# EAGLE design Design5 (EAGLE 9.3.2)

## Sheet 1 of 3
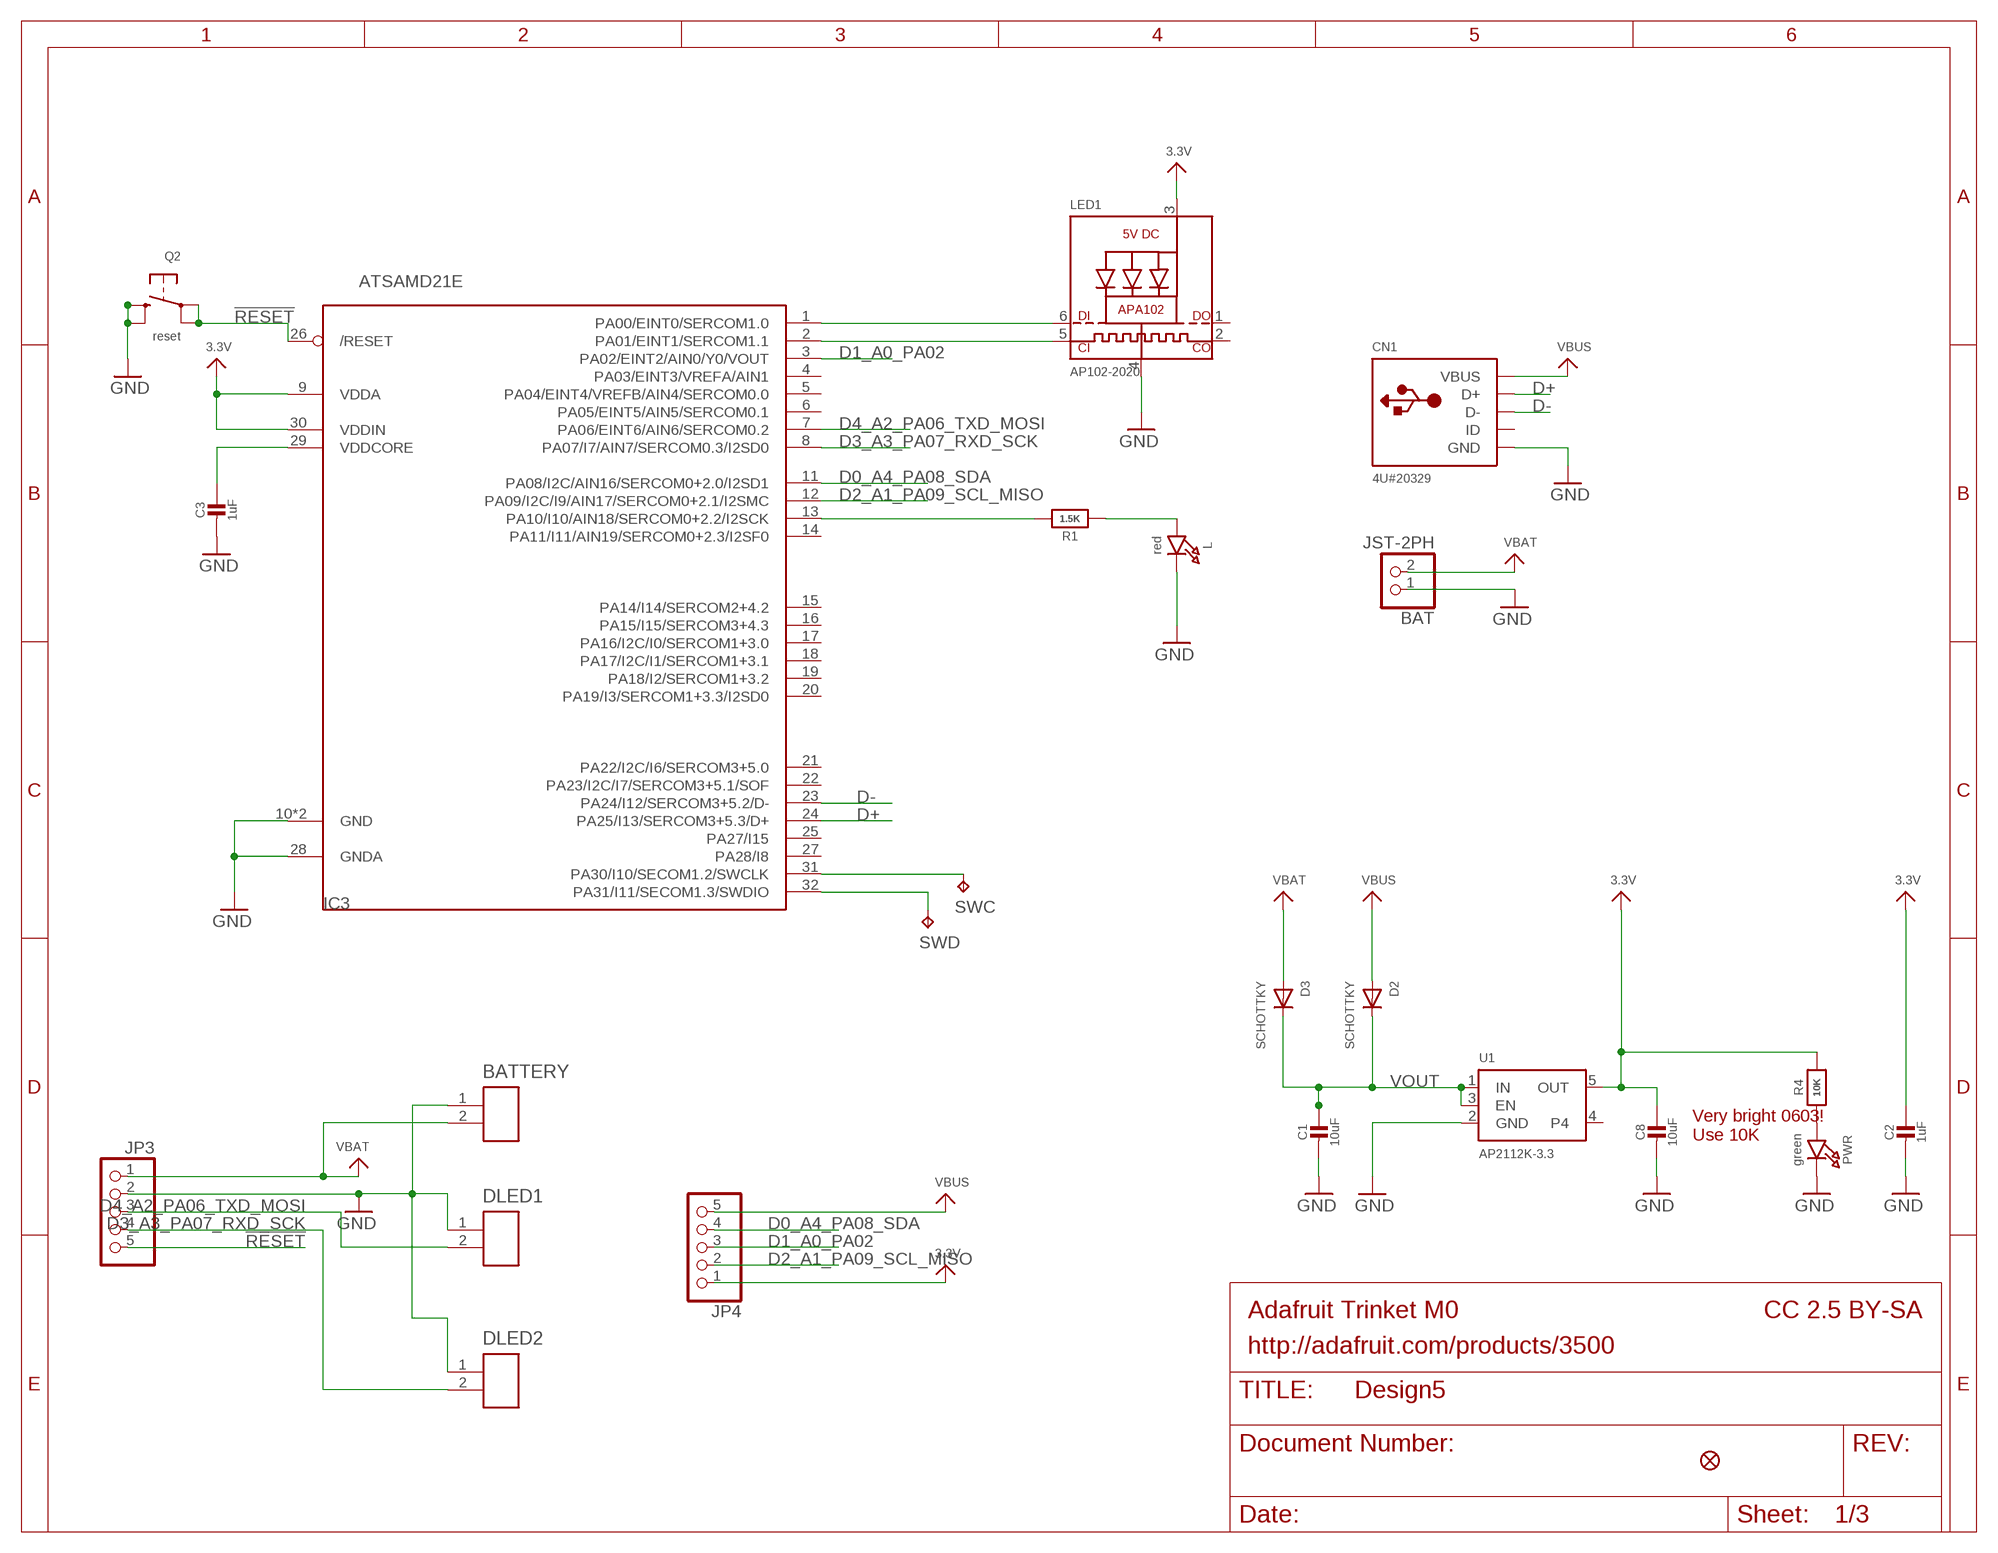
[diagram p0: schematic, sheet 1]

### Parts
BAT  JST-2PH  CON_JST_PH_2PIN  [JSTPH2]
BATTERY  JST_ZH_2PIN  [JST_ZH_2PIN]
C1  10uF  CAP_CERAMIC0805-NOOUTLINE  [0805-NO]
C2  1uF  CAP_CERAMIC0603_NO  [0603-NO]
C3  1uF  CAP_CERAMIC0603_NO  [0603-NO]
C8  10uF  CAP_CERAMIC0805-NOOUTLINE  [0805-NO]
CN1  4U#20329  USB_MICRO_20329_V2  [4UCONN_20329_V2]
D2  SCHOTTKY  DIODE_SOD-123FL  [SOD-123FL]
D3  SCHOTTKY  DIODE_SOD-123FL  [SOD-123FL]
DLED1  JST_ZH_2PIN  [JST_ZH_2PIN]
DLED2  JST_ZH_2PIN  [JST_ZH_2PIN]
IC3  ATSAMD21E  [QFN32_5MM]
JP3  HEADER-1X576MIL  [1X05_ROUND_76]
JP4  HEADER-1X576MIL  [1X05_ROUND_76]
L  red  LED0603_NOOUTLINE  [CHIPLED_0603_NOOUTLINE]
LED1  AP102-2020  APA1022020  [APA102_2020]
PWR  green  LED0603_NOOUTLINE  [CHIPLED_0603_NOOUTLINE]
Q2  reset  SWITCH_TACT_SMT4.6X2.8  [BTN_KMR2_4.6X2.8]
R1  1.5K  RESISTOR_0603_NOOUT  [0603-NO]
R4  10K  RESISTOR_0603_NOOUT  [0603-NO]
SWC  TPB1,27  [B1,27]
SWD  TPB1,27  [B1,27]
U1  AP2112K-3.3  VREG_SOT23-5  [SOT23-5]
U$6  FIDUCIAL_1MM  [FIDUCIAL_1MM]

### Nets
3.3V: C2.1 C8.1 IC3.9(VDDA) IC3.30(VDDIN) JP4.1 LED1.3(VDD) R4.2 U1.5(OUT) ; also sheet 2,3
!RESET: IC3.26(/RESET) JP3.5 Q2.A'(P1) Q2.A(P)
A3: IC3.1(PA00/EINT0/SERCOM1.0) LED1.6(DI)
D0_A4_PA08_SDA: IC3.11(PA08/I2C/AIN16/SERCOM0+2.0/I2SD1) JP4.4
D1_A0_PA02: IC3.3(PA02/EINT2/AIN0/Y0/VOUT) JP4.3 ; also sheet 2
D2_A1_PA09_SCL_MISO: IC3.12(PA09/I2C/I9/AIN17/SERCOM0+2.1/I2SMC) JP4.2 ; also sheet 3
D3_A3_PA07_RXD_SCK: DLED2.2 IC3.8(PA07/I7/AIN7/SERCOM0.3/I2SD0) JP3.4
D4_A2_PA06_TXD_MOSI: DLED1.2 IC3.7(PA06/EINT6/AIN6/SERCOM0.2) JP3.3
D+: CN1.D+ IC3.24(PA25/I13/SERCOM3+5.3/D+)
D-: CN1.D- IC3.23(PA24/I12/SERCOM3+5.2/D-)
GND: BAT.1 BATTERY.1 C1.2 C2.2 C3.2 C8.2 CN1.BASE@1(GND) CN1.BASE@2(GND) CN1.GND CN1.SPRT@1(GND) CN1.SPRT@2(GND) CN1.SPRT@3(GND) CN1.SPRT@4(GND) DLED1.1 DLED2.1 IC3.10(GND) IC3.28(GNDA) IC3.33(GND) JP3.2 L.C LED1.4(GND) PWR.C Q2.B'(S1) Q2.B(S) U1.2(GND) ; also sheet 2,3
N$1: L.A R1.1
N$2: IC3.13(PA10/I10/AIN18/SERCOM0+2.2/I2SCK) R1.2
N$3: IC3.31(PA30/I10/SECOM1.2/SWCLK) SWC.TP
N$4: IC3.32(PA31/I11/SECOM1.3/SWDIO) SWD.TP
N$6: PWR.A R4.1
N$8: IC3.2(PA01/EINT1/SERCOM1.1) LED1.5(CKI)
VBAT: BAT.2 BATTERY.2 D3.A JP3.1
VBUS: CN1.VBUS D2.A JP4.5
VDDCORE: C3.1 IC3.29(VDDCORE)
VOUT: C1.1 D2.C D3.C U1.1(IN) U1.3(EN)
Unconnected: CN1.ID IC3.4(PA03/EINT3/VREFA/AIN1) IC3.5(PA04/EINT4/VREFB/AIN4/SERCOM0.0) IC3.6(PA05/EINT5/AIN5/SERCOM0.1) IC3.14(PA11/I11/AIN19/SERCOM0+2.3/I2SF0) IC3.15(PA14/I14/SERCOM2+4.2) IC3.16(PA15/I15/SERCOM3+4.3) IC3.17(PA16/I2C/I0/SERCOM1+3.0) IC3.18(PA17/I2C/I1/SERCOM1+3.1) IC3.19(PA18/I2/SERCOM1+3.2) IC3.20(PA19/I3/SERCOM1+3.3/I2SD0) IC3.21(PA22/I2C/I6/SERCOM3+5.0) IC3.22(PA23/I2C/I7/SERCOM3+5.1/SOF) IC3.25(PA27/I15) IC3.27(PA28/I8) LED1.1(DO) LED1.2(CKO) U1.4

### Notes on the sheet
- Very bright 0603!
  Use 10K
- Adafruit Trinket M0 | CC 2.5 BY-SA
- http://adafruit.com/products/3500

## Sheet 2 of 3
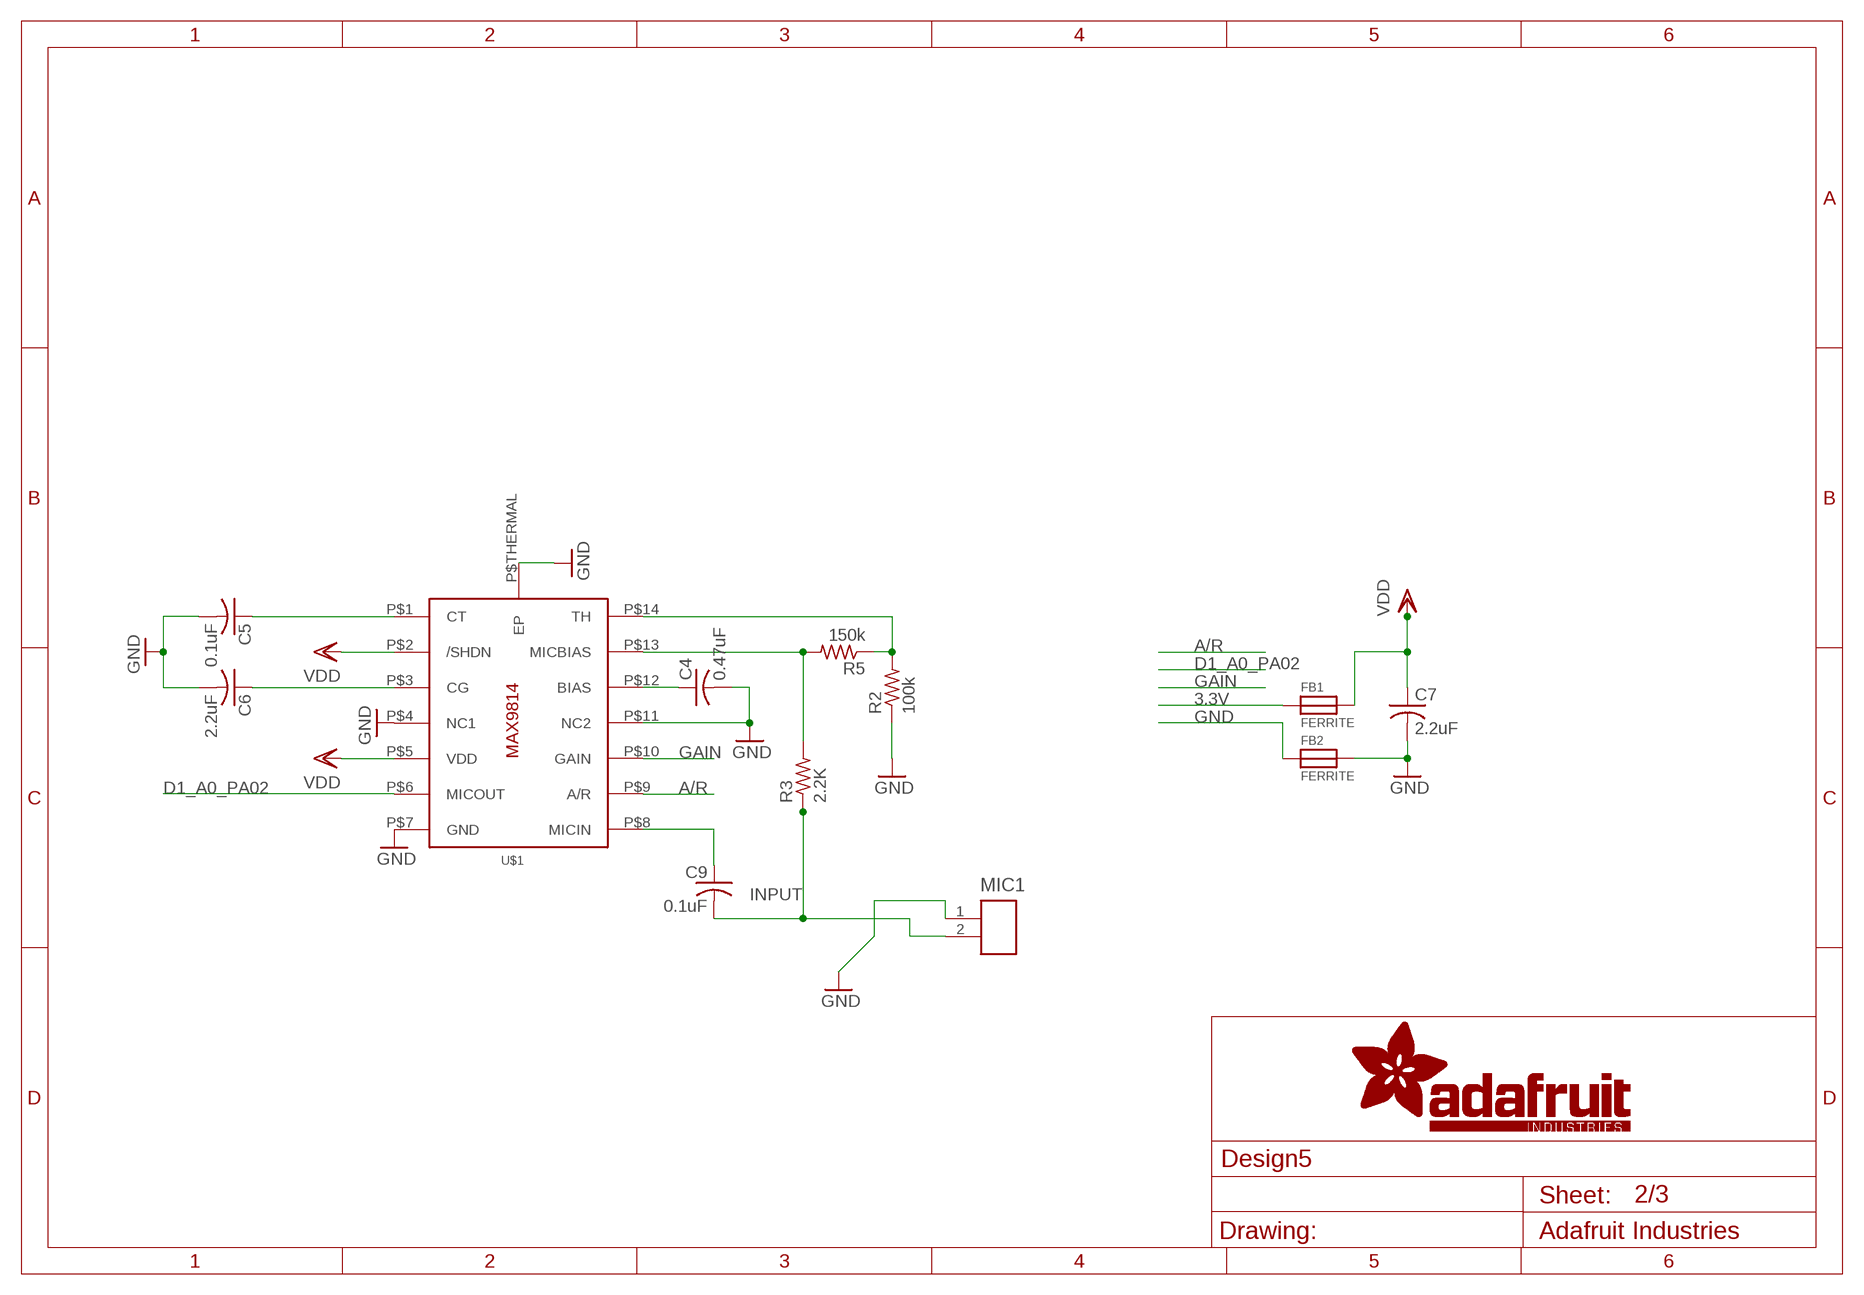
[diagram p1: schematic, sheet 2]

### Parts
C4  0.47uF  C-USC0805K  [C0805K]
C5  0.1uF  C-USC0805K  [C0805K]
C6  2.2uF  C-USC0805K  [C0805K]
C7  2.2uF  C-USC0805K  [C0805K]
C9  0.1uF  C-USC0805K  [C0805K]
FB1  FERRITE  FERRITE0805  [0805]
FB2  FERRITE  FERRITE0805  [0805]
MIC1  JST_ZH_2PIN  [JST_ZH_2PIN]
R2  100k  R-US_R0805  [R0805]
R3  2.2K  R-US_R0805  [R0805]
R5  150k  R-US_R0805  [R0805]
U$1  MAX9814TDFN14  [TDFN14_3X3MM]

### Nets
3.3V: FB1.1 ; also sheet 1,3
A/R: U$1.P$9(A/R)
D1_A0_PA02: U$1.P$6(MICOUT) ; also sheet 1
GAIN: U$1.P$10(GAIN)
GND: C4.2 C5.2 C6.2 C7.2 FB2.1 FB2.2 MIC1.1 R2.1 U$1.P$4(NC1) U$1.P$7(GND) U$1.P$11(NC2) U$1.P$THERMAL(EP) ; also sheet 1,3
INPUT: C9.2 MIC1.2 R3.1
N$5: C9.1 U$1.P$8(MICIN)
N$7: C4.1 U$1.P$12(BIAS)
N$9: C5.1 U$1.P$1(CT)
N$10: C6.1 U$1.P$3(CG)
N$11: R2.2 R5.1 U$1.P$14(TH)
N$12: R3.2 R5.2 U$1.P$13(MICBIAS)
VDD: C7.1 FB1.2 U$1.P$2(/SHDN) U$1.P$5(VDD) ; also sheet 3

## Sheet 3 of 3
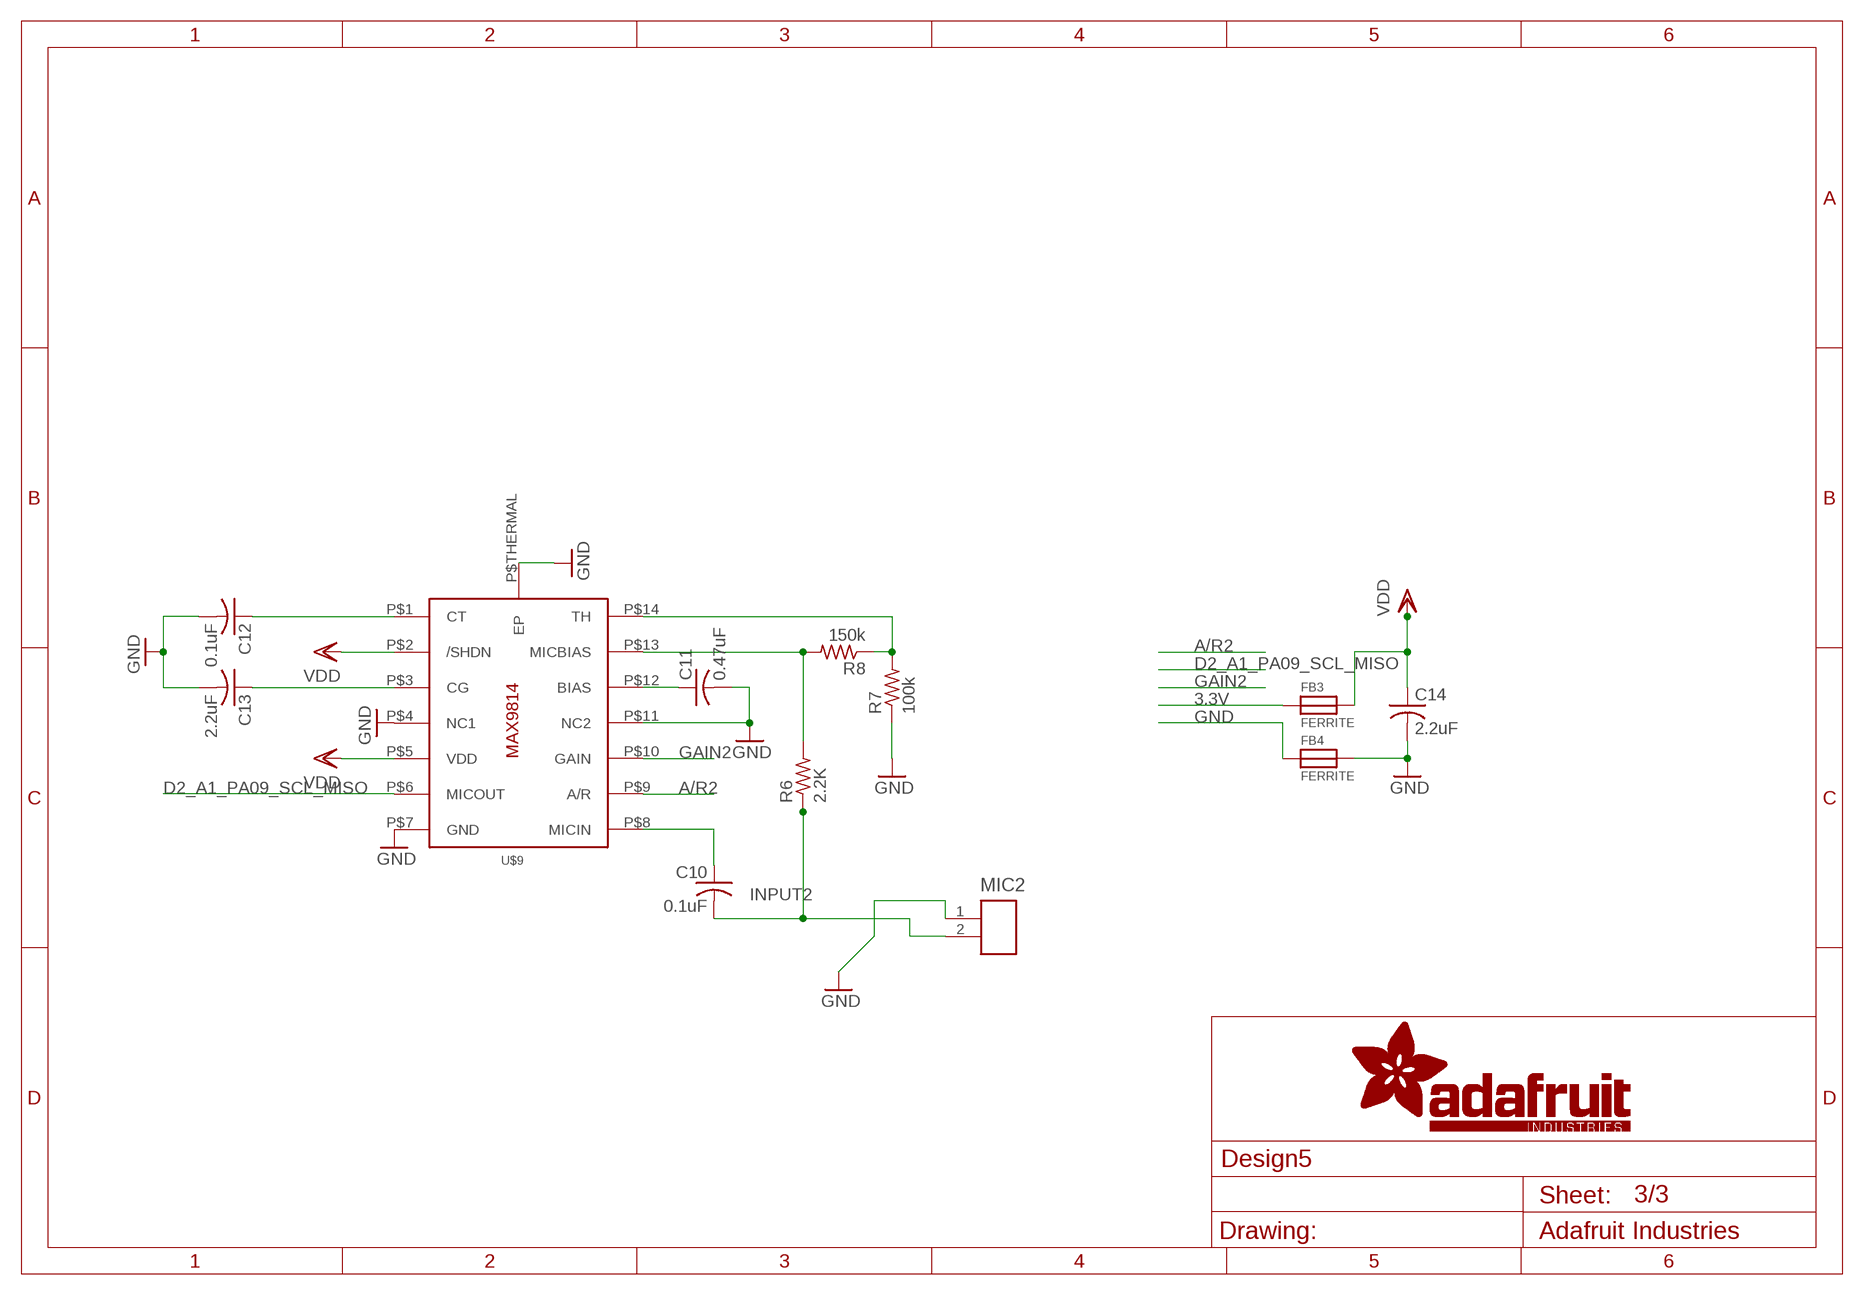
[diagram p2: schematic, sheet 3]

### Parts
C10  0.1uF  C-USC0805K  [C0805K]
C11  0.47uF  C-USC0805K  [C0805K]
C12  0.1uF  C-USC0805K  [C0805K]
C13  2.2uF  C-USC0805K  [C0805K]
C14  2.2uF  C-USC0805K  [C0805K]
FB3  FERRITE  FERRITE0805  [0805]
FB4  FERRITE  FERRITE0805  [0805]
MIC2  JST_ZH_2PIN  [JST_ZH_2PIN]
R6  2.2K  R-US_R0805  [R0805]
R7  100k  R-US_R0805  [R0805]
R8  150k  R-US_R0805  [R0805]
U$9  MAX9814TDFN14  [TDFN14_3X3MM]

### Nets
3.3V: FB3.1 ; also sheet 1,2
A/R2: U$9.P$9(A/R)
D2_A1_PA09_SCL_MISO: U$9.P$6(MICOUT) ; also sheet 1
GAIN2: U$9.P$10(GAIN)
GND: C11.2 C12.2 C13.2 C14.2 FB4.1 FB4.2 MIC2.1 R7.1 U$9.P$4(NC1) U$9.P$7(GND) U$9.P$11(NC2) U$9.P$THERMAL(EP) ; also sheet 1,2
INPUT2: C10.2 MIC2.2 R6.1
N$13: C11.1 U$9.P$12(BIAS)
N$14: C10.1 U$9.P$8(MICIN)
N$15: C12.1 U$9.P$1(CT)
N$16: C13.1 U$9.P$3(CG)
N$17: R7.2 R8.1 U$9.P$14(TH)
N$18: R6.2 R8.2 U$9.P$13(MICBIAS)
VDD: C14.1 FB3.2 U$9.P$2(/SHDN) U$9.P$5(VDD) ; also sheet 2

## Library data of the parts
BAT = microbuilder:CON_JST_PH_2PIN: JST 2-Pin Right-Angle Connector
BATTERY DLED1 DLED2 MIC1 MIC2 = kanflo:JST_ZH_2PIN: JST ZH connector, 2 pins
C1-C3 C8 = microbuilder:CAP_CERAMIC: Ceramic Capacitors
C4-C7 C9-C14 = adafruit:C-US: CAPACITOR, American symbol
CN1 = microbuilder:USB: USB Connectors USBMINIB - Surface Mount Female Mini-B USB Connector 4UConnector: 06564
D2 D3 = adafruit:DIODE: Diode
FB1-FB4 = microbuilder:FERRITE: Ferrite Bead
IC3 = microbuilder:ATSAMD21E
JP3 JP4 = microbuilder:HEADER-1X5: PIN HEADER
L PWR = microbuilder:LED: LED
LED1 = microbuilder:APA102: APA102/DotStar Pixels VCC: 5V DC Refresh Rate: 400Hz
Q2 = microbuilder:SWITCH_TACT_SMT: SMT Tact Switches 6x6mm - Digikey: P12940SCT-ND KMR2 (4.6x2.8mm) - Digikey: 401-1426-1-ND EVQ-PQHB55 - Light Touch, 160GF (4.5x4.5mm) - Digikey: P8090SCT-ND KMT0 - KMT021 NGJ LHS (etc.) IP68/Waterproof - Digikey: CKN10289CT-ND
R1 R4 = microbuilder:RESISTOR: Resistors
R2 R3 R5-R8 = adafruit:R-US_: RESISTOR, American symbol
SWC SWD = testpad:TP: Test pad
U1 = microbuilder:VREG_SOT23-5: SOT23-5 Fixed Voltage Regulators Part Current Out V Out V In V Dropout θJA (°C/W) TJ (°C) Digikey Part No. ADP121 150mA 3.3V 3.4-5.5V 0.09V @ 150mA -- -- ADP121-AUJZ33R7CT-ND ADP121 150mA 3.0V 3.1-5.5V 0.09V @ 150mA -- -- ADP121-AUJZ30R7CT-ND ADP122 300mA 3.3V 3.4-5.5V 0.085V @ 300mA -- --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
U$1 U$9 = adafruit:MAX9814
U$6 = microbuilder:FIDUCIAL: Fiducial Alignment Points; BOM: EXCLUDE

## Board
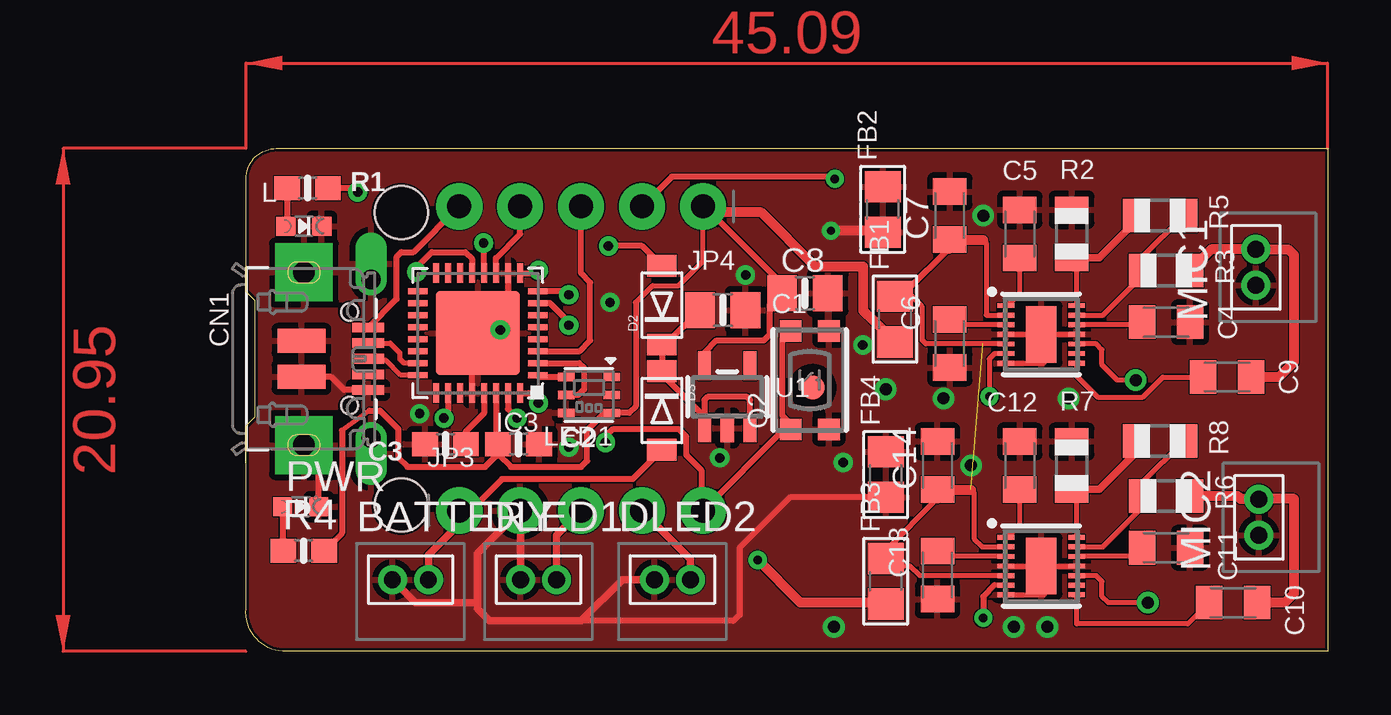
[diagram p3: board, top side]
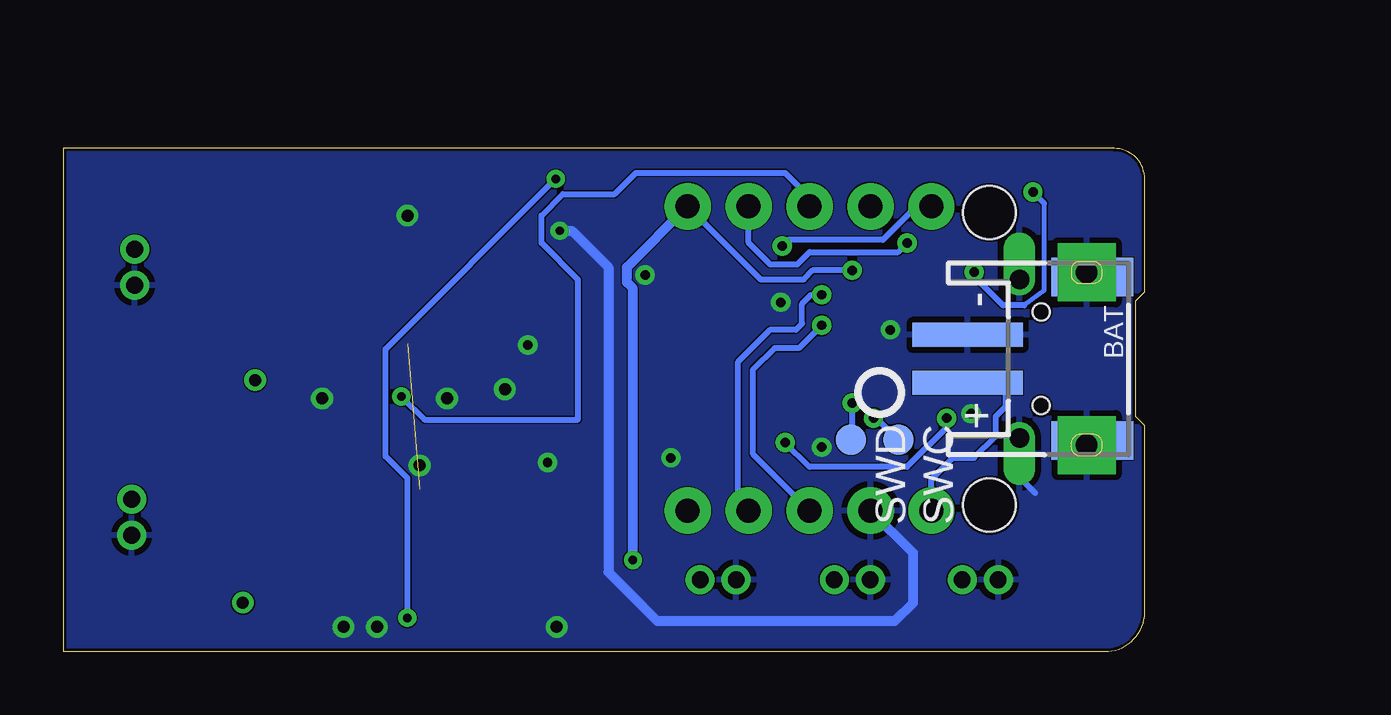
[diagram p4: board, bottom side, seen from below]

Size 45.09 x 20.95 mm. Coordinates in mm from the lower left corner, seen from the top.
Outline: 1.27,20.95 45.09,20.95 45.09,0 1.53,0 arc-90 0,1.78 0,9.4 0.39,9.78 0.39,14.61 0,14.99 0,19.68 arc-90 1.27,20.95
Copper layers (1*16): Top 0.035mm / dielectric 1.5mm / Bottom 0.035mm
Design rules "default *": minimum track width 6mil, minimum drill 0.35mm, track to track 2mil, track to pad 2mil, pad to pad 2mil, via to via 2mil, smd to smd 6mil, copper to edge 5mil, drill to drill 6mil, minimum pad ring 10mil, minimum via ring 8mil, stop-mask expansion 4mil, vias tented up to drill 0mil, thermal gap 10mil
Holes 2.2 mm at 6.48,6.1 6.48,18.29

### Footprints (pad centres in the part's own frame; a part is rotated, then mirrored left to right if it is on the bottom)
JSTPH2 = smd 1 x 4.6: 1 -1,-3.7; 2 1,-3.7 | smd 1.6 x 3.4: NC1 -3.4,1.5; NC2 3.4,1.5
JST_ZH_2PIN = drill 0.7 pad 1: 1 -0.75,0.45; 2 0.75,0.45
0805-NO = smd 1.24 x 1.5: 1 -0.95,0; 2 0.95,0
0603-NO = smd 1.075 x 1: 1 -0.85,0; 2 0.85,0
C0805K = smd 1.1 x 1.4: 1 -1,0; 2 1,0
4UCONN_20329_V2 = smd 1 x 2: BASE@1 -0.75,-2; BASE@2 0.75,-2 | smd 0.4 x 1.35: D+ 0,0.775; D- -0.65,0.775; GND 1.3,0.775; ID 0.65,0.775; VBUS -1.3,0.775 | drill 0.8 pad 1.143 offset: SPRT@1 -3.3,0.9; SPRT@2 3.3,0.9 | drill 0.9 pad 2.413 square: SPRT@3 -3.6,-1.9; SPRT@4 3.6,-1.9 | hole 0.7: -1.95,0; 1.95,0
SOD-123FL = smd 0.91 x 1.22: A 1.637,0; C -1.637,0
0805 = smd 1.3 x 1.5: 1 -0.95,0; 2 0.95,0
QFN32_5MM = smd 0.8 x 0.25: 1 -2.5,1.75; 2 -2.5,1.25; 3 -2.5,0.75; 4 -2.5,0.25; 5 -2.5,-0.25; 6 -2.5,-0.75; 7 -2.5,-1.25; 8 -2.5,-1.75; 17 2.5,-1.75; 18 2.5,-1.25; 19 2.5,-0.75; 20 2.5,-0.25; 21 2.5,0.25; 22 2.5,0.75; 23 2.5,1.25; 24 2.5,1.75 | smd 0.25 x 0.8: 9 -1.75,-2.5; 10 -1.25,-2.5; 11 -0.75,-2.5; 12 -0.25,-2.5; 13 0.25,-2.5; 14 0.75,-2.5; 15 1.25,-2.5; 16 1.75,-2.5; 25 1.75,2.5; 26 1.25,2.5; 27 0.75,2.5; 28 0.25,2.5; 29 -0.25,2.5; 30 -0.75,2.5; 31 -1.25,2.5; 32 -1.75,2.5 | smd 3.5 x 3.5: 33 0,0
1X05_ROUND_76 = drill 1 pad 1.93: 1 -5.08,0; 2 -2.54,0; 3 0,0; 4 2.54,0; 5 5.08,0
CHIPLED_0603_NOOUTLINE = smd 0.8 x 0.8: A 0,-0.75; C 0,0.75
APA102_2020 = smd 0.7 x 0.35: 1 -0.95,-0.75; 2 -0.95,0; 3 -0.95,0.75; 4 0.95,0.75; 5 0.95,0; 6 0.95,-0.75
BTN_KMR2_4.6X2.8 = smd 0.9 x 0.9: A 2.05,0.8; A' -2.05,0.8; B 2.05,-0.8; B' -2.05,-0.8
R0805 = smd 1.1 x 1.4: 1 -1,0; 2 1,0
B1,27 = smd 1.27 x 1.27: TP 0,0
SOT23-5 = smd 0.55 x 1.2: 1 -0.95,-1.3; 2 0,-1.3; 3 0.95,-1.3; 4 0.95,1.3; 5 -0.95,1.3
TDFN14_3X3MM = smd 0.7 x 0.2: P$1 -1.475,1.2; P$2 -1.475,0.8; P$3 -1.475,0.4; P$4 -1.475,0; P$5 -1.475,-0.4; P$6 -1.475,-0.8; P$7 -1.475,-1.2; P$8 1.475,-1.2; P$9 1.475,-0.8; P$10 1.475,-0.4; P$11 1.475,0; P$12 1.475,0.4; P$13 1.475,0.8; P$14 1.475,1.2 | smd 1.27 x 2.35: P$THERMAL 0,0
FIDUCIAL_1MM = smd 1 x 1: 1 0,0

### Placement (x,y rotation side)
BAT  3.69,12.19 270 bottom
BATTERY  6.86,2.54 0 top
C1  19.88,14.22 0 top
C2  11.37,8.64 0 top
C3  8.32,8.64 180 top
C4  38.36,13.72 0 top
C5  32.26,17.4 90 top
C6  29.34,12.83 270 top
C7  29.34,18.16 90 top
C8  23.31,14.92 0 top
C9  40.9,11.43 0 top
C10  41.15,2.03 0 top
C11  38.36,4.32 0 top
C12  32.26,7.75 90 top
C13  28.83,3.17 270 top
C14  28.83,7.75 90 top
CN1  4.32,12.19 270 top
D2  17.34,14.43 90 top
D3  17.34,10.03 270 top
DLED1  12.2,2.54 0 top
DLED2  17.78,2.54 0 top
FB1  27.06,13.84 90 top
FB2  26.55,18.41 90 top
FB3  26.67,2.92 90 top
FB4  26.67,7.37 90 top
IC3  9.67,13.26 180 top
JP3  13.97,5.87 0 top
JP4  13.97,18.54 180 top
L  2.42,17.72 270 top
LED1  14.3,10.69 180 top
MIC1  42.55,16 90 top
MIC2  42.68,5.59 90 top
PWR  2.29,6.03 270 top
Q2  23.5,11.3 90 top
R1  2.57,19.3 0 top
R2  34.42,17.4 270 top
R3  38.36,15.88 180 top
R4  2.42,4.19 0 top
R5  38.1,18.16 0 top
R6  38.36,6.48 180 top
R7  34.42,7.75 270 top
R8  38.1,8.76 0 top
SWC  10.27,8.83 270 bottom
SWD  12.26,8.83 270 bottom
U1  20.07,10.6 0 top
U$1  33.15,13.21 0 top
U$6  23.63,10.99 90 top
U$9  33.15,3.56 0 top
U$12  [PCBFEAT-REV-040]  11.05,10.79 0 bottom

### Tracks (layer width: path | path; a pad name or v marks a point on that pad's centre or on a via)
3.3V  (via drill 0.35, 0.39)
  Top 0.203: 5.15,10.03 4,9.2 | 16.26,14.54 16.96,15.24 18.04,15.24 19.05,16.26 19.05,18.29 JP4.1
  Top 0.254: C2.1 10.52,8.22 11.05,7.68 13.97,7.68 14.23,7.94 14.23,9.21 14.96,9.94 LED1.3 15.98,9.94 16.26,10.22 16.26,14.54 | JP4.1 19.12,18.54 22.36,15.3 C8.1 22.29,14.92 21.85,14.48 21.85,13.21 21.59,12.95 19.63,12.95 19.12,12.45 U1.5 | 5.15,10.03 5.59,10.03 6.35,9.27 6.35,8.06 6.74,7.68 9.97,7.68 10.42,8.13 10.42,8.53 C2.1 | IC3.9 12.09,15.76 v12.2,15.88 | IC3.30 10.42,8.73 C2.1 | R4.2 4,4.93 4,9.2
  Top 0.406: FB1.1 26.16,13.79 25.74,14.2 25.74,16.03 23.75,16.03 21.49,18.29 19.05,18.29 | FB3.1 26.67,2.03 23.12,2.03 v21.34,3.81
  Bottom 0.254: v12.2,15.88 13.85,15.88 14.23,15.49 16.01,15.49 JP4.1
  Bottom 0.406: v21.34,3.81 21.34,15.12 21.59,15.37 21.59,16.01 JP4.1
!RESET  (via drill 0.39)
  Top 0.254: Q2.A 22.36,13 22.36,9.84 22.7,9.49 Q2.A' 22.44,9.25 JP3.5 18.99,5.93 18.99,7.56 18.36,8.19 18.36,8.95 18.04,9.27 15.31,9.27 14.99,8.95 v14.99,8.7 | IC3.26 8.42,9.81 arc-90 v8.26,9.71
  Bottom 0.254: v8.26,9.71 8.26,9.33 9.91,7.68 13.97,7.68 v14.99,8.7
A3
  Top 0.254: IC3.1 12.25,11.44 LED1.6
D0_A4_PA08_SDA
  Top 0.254: IC3.11 10.42,16.39 11.43,17.4 JP4.4
D1_A0_PA02  (via drill 0.35)
  Top 0.203: U$1.P$6 31.21,12.41 30.99,12.19 30.99,10.92
  Top 0.254: IC3.3 13.92,12.51 14.36,12.95 14.36,15.37 13.97,15.75 JP4.3 | 30.99,10.92 v30.99,10.62
  Bottom 0.254: v30.99,10.62 30.02,9.65 23.63,9.65 23.63,15.49 25.15,17.02 25.15,18.16 24.26,19.05 22.1,19.05 21.21,19.94 14.99,19.94 13.97,18.92 JP4.3
D2_A1_PA09_SCL_MISO  (via drill 0.35, 0.39)
  Top 0.203: U$9.P$6 31.21,2.76
  Top 0.254: IC3.12 9.92,17.01 v9.91,17.02 | 31.21,2.76 30.74,2.29 v30.74,1.39 | v24.55,19.69 24.45,19.79 17.76,19.79 JP4.2
  Bottom 0.254: JP4.2 16.51,17.02 15.63,16.13 14.48,16.13 13.97,16.64 10.29,16.64 v9.91,17.02 | v30.74,1.39 30.74,7.22 31.65,8.13 31.65,12.59 v24.55,19.69
D3_A3_PA07_RXD_SCK  (via drill 0.39)
  Top 0.254: v13.47,14.86 13.31,15.01 IC3.8
  Top 0.305: DLED2.2 18.53,3.85 JP3.4
  Bottom 0.254: JP3.4 16.96,6.31 16.96,12.06 15.63,13.4 14.55,13.4 14.29,13.65 14.29,14.48 13.91,14.86 v13.47,14.86
D4_A2_PA06_TXD_MOSI  (via drill 0.39)
  Top 0.254: v13.47,13.59 13.47,13.72 12.68,14.51 IC3.7
  Top 0.305: DLED1.2 12.95,4.84 JP3.3
  Bottom 0.254: JP3.3 16.32,8.22 16.32,11.75 15.43,12.64 14.42,12.64 v13.47,13.59
D+
  Top 0.203: IC3.24 6.46,11.51 5.85,12.13 5.16,12.13
  Top 0.254: 5.16,12.13 CN1.D+
D-
  Top 0.203: CN1.D- 6.02,12.84 6.42,12.45 6.42,12.19 6.6,12.01 IC3.23
GAIN  (via drill 0.5)
  Top 0.203: U$1.P$10 35.46,12.81 35.69,12.57 35.69,11.94 36.33,11.3 v37.09,11.3
GAIN2  (via drill 0.5)
  Top 0.203: U$9.P$10 35.46,3.16 35.69,2.92 35.69,2.29 35.95,2.03 v37.6,2.03
GND  (via drill 0.35, 0.39, 0.5)
  Top 0.203: U$1.P$4 33.28,13.21 | 33.28,13.21 U$1.P$11 | U$1.P$7 33.28,12.01 33.28,13.21 | U$9.P$4 33.28,3.56 | 33.28,3.56 U$9.P$11 | U$9.P$7 33.28,2.36 33.28,3.56
  Top 0.254: CN1.GND 4.1,10.89 3.55,11.44 CN1.BASE@2 | IC3.28 9.42,13.01 arc-90 IC3.33 10.47,13.26 v10.61,13.4 arc90 10.92,13.71 IC3.10 | PWR.C 3.04,7.97 CN1.SPRT@4 | FB4.1 22.68,6.42 20.58,4.32 20.58,1.52 20.32,1.27 13.72,1.27
  Top 0.305: DLED2.1 15.69,2.99 13.97,1.27 13.72,1.27 10.16,1.27 9.66,1.78 9.66,2.03 | 9.66,2.03 9.66,4.09 JP3.2 11.45,5.85 DLED1.1 | BATTERY.1 7.07,2.03 9.66,2.03
  Top 0.406: FB2.1 26.49,17.53 v24.39,17.53
  Bottom 0.254: CN1.SPRT@2 5.22,7.25 4.58,6.6
  Bottom 0.406: v24.39,17.53 23.88,17.53 22.36,16 22.36,3.3 20.32,1.27 10.42,1.27 9.66,2.03 9.66,4.09 JP3.2
  other vias: 24.9,7.87 19.75,8.06 20.83,15.68 25.72,12.76 13.47,8.51 7.24,9.91 15.18,14.54 29.09,10.54 30.74,18.16 34.29,10.54 26.67,10.92 32.01,1.02 30.23,7.75 33.41,1.02 24.52,1.02
  pour Bottom: 0,0 45.09,0 45.09,20.95 0,20.95
  pour Top: 0,20.95 0,0 45.09,0 45.09,20.95
INPUT
  Top 0.406: R3.1 40.24,16.75 MIC1.2 43.45,16.75 43.69,16.51 43.69,12.06 43.06,11.43 C9.2
INPUT2
  Top 0.406: R6.1 41.34,6.48 41.47,6.35 42.24,6.35 | 42.24,6.35 43.69,6.35 43.69,2.41 43.31,2.03 C10.2 | 42.24,6.35 MIC2.2
N$1
  Top 0.254: R1.1 1.72,17.77 L.A
N$2  (via drill 0.39)
  Top 0.254: IC3.13 9.42,16.36 9.15,16.64 7.75,16.64 7.12,16 v7.12,15.81 | v4.67,19.14 4.5,19.3 R1.2
  Bottom 0.203: 5.03,14.41 4.2,15.05 4.2,18.67
  Bottom 0.254: 5.03,14.41 5.91,14.41 7.12,15.62 v7.12,15.81 | 4.2,18.67 v4.67,19.14
N$3  (via drill 0.39)
  Top 0.254: IC3.31 10.92,10.1 v11.31,9.71
  Bottom 0.254: SWC.TP 10.29,8.83 11.18,9.71 11.22,9.71 v11.31,9.71
N$4  (via drill 0.39)
  Top 0.254: IC3.32 11.78,10.76 v12.2,10.35
  Bottom 0.254: SWD.TP 12.2,8.89 v12.2,10.35
N$5
  Top 0.203: U$1.P$8 34.63,11.48 35.51,10.6 37.38,10.6 38.22,11.43 C9.1
N$6
  Top 0.254: PWR.A 1.54,4.22 R4.1
N$7
  Top 0.203: U$1.P$12 37.25,13.61 C4.1
N$8
  Top 0.254: LED1.5 13.87,10.69 14.1,10.92 14.1,11.81 13.9,12.01 IC3.2
N$9
  Top 0.203: C5.1 32.26,14.92 31.75,14.41 U$1.P$1
N$10
  Top 0.203: U$1.P$3 29.25,13.61
  Top 0.254: C6.1 29.25,13.83 29.25,13.61
N$11
  Top 0.203: R2.2 34.31,16.4 34.29,16.38 34.65,16.03 34.63,16 U$1.P$14
  Top 0.254: 37.1,17.92 R5.1
  Top 0.305: R2.2 35.58,16.4 37.1,17.92
N$12
  Top 0.203: U$1.P$13 35.73,14.01 37.36,15.64 R3.2 37.36,16.41 R5.2
N$13
  Top 0.203: U$9.P$12 37,3.96 C11.1
N$14
  Top 0.203: U$9.P$8 34.63,1.14 39.26,1.14 C10.1
N$15
  Top 0.203: C12.1 32.26,5.27 31.75,4.76 U$9.P$1
N$16
  Top 0.203: U$9.P$3 29.25,3.96
  Top 0.254: C13.1 29.25,4.17 29.25,3.96
N$17
  Top 0.203: R7.2 34.31,6.75 34.29,6.73 34.65,6.37 34.63,6.35 U$9.P$14
  Top 0.254: 37.1,8.27 R8.1
  Top 0.305: R7.2 35.58,6.75 37.1,8.27
N$18
  Top 0.203: U$9.P$13 35.73,4.36 37.36,5.99 R6.2 37.36,7.02 R8.2
VBAT
  Top 0.254: JP3.1 9.36,5.87 10.67,7.18 16.12,7.18 D3.A
  Top 0.305: BATTERY.2 7.61,4.02 8.75,5.16 8.75,5.72 JP3.1
  Bottom 0.254: JP3.1 8.89,7.18 8.01,8.06 7.12,8.06 6.21,8.97 6.21,9.79 5.78,10.22 5.78,11.18 5.8,11.19 BAT.2
VBUS  (via drill 0.39)
  Top 0.254: CN1.VBUS 6.29,14.69 6.29,16.45 6.48,16.64 6.99,16.64 JP4.5 | D2.A 16.51,16.89 v15.12,16.89
  Bottom 0.254: JP4.5 9.53,18.54 10.93,17.14 14.86,17.14 v15.12,16.89
VDD  (1 unrouted)
  Top 0.203: U$1.P$2 30.87,14.01 30.87,17.02 30.74,17.14 30.72,17.16 | 30.72,12.81 U$1.P$5 28.34,12.81 28.2,12.95 28.2,14.35 27.53,15.02 | U$9.P$2 30.7,4.36 30.36,4.7 30.36,6.6 30.23,6.73 30.21,6.75 | 30.72,3.16 U$9.P$5 28.09,3.16 27.69,3.56 26.99,3.56 FB3.2 26.67,4.21 28.83,6.37
  Top 0.254: FB1.2 27.06,14.73 27.25,14.73 27.53,15.02 29.34,16.82 C7.1 | 28.83,6.67 C14.1
  Top 0.406: 30.74,17.14 29.34,17.14 C7.1 29.34,16.79 29.19,16.79 29.09,16.89 | 30.23,6.73 28.83,6.73 C14.1 28.83,6.37 28.68,6.37 28.58,6.48
VDDCORE
  Top 0.254: IC3.29 9.92,9.92 9.17,9.17 C3.1
VOUT
  Top 0.203: D2.C 17.5,12.79
  Top 0.254: U1.3 21.02,10.48 20.9,10.6 19.24,10.6 19.12,10.48 U1.1 19.12,9.78 17.23,11.67 D3.C D2.C | 17.5,12.79 C1.1
(copper drawn outside any net)
  shapes: Top area x2

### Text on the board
bPlace: - | +
tDocu: D0/A4/SDA | D1/A0/VOUT | D2/A1/SCL/MISO

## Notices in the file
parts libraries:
microbuilder: This work is placed in the public domain, and may be freely used for commercial and non-commercial work with the following conditions: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
